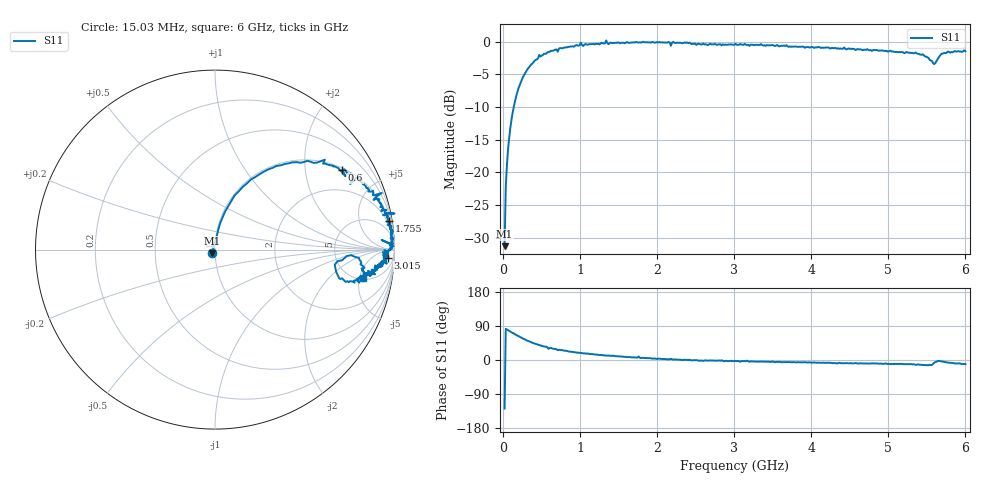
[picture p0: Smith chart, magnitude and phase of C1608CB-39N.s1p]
!	Network	Analyzer	HP8753E.07.74:	Oct	30	2002	Serial	No.	JP38451487
!	Hewlett-Packard
!	7	Sep	2009	9:44:38
!	Frequency	S11
#	HZ	S	RI	R	50
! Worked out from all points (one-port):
!   400 points, 15.03 MHz to 6 GHz, reference 50 ohm
!   lowest |S11| = -31.3 dB at 15.03 MHz (marker M1), VSWR 1.06, Z = 48.3 - j2.08 ohm
!   |S11| at or under -10 dB: start of sweep to 133.9 MHz
!   S11 on the Smith chart (normalised r, x): 15.03 MHz: 0.97, -0.04; 600 MHz: 1.07, +3.15; 1.755 GHz: 1, +12; 3.015 GHz: 20, -26; 6 GHz: 5.27, -5.76
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1.502992e7  -0.0168 -0.0215
3.002985e7  0.0105 0.0768
6.00297e7  0.0293 0.148
1.500292e8  0.132 0.324
3.150284e8  0.392 0.478
4.650277e8  0.612 0.501
6.00027e8  0.709 0.444
7.650262e8  0.798 0.389
1.005025e9  0.929 0.316
1.245024e9  0.926 0.214
1.335023e9  1 0.201
1.365023e9  0.936 0.192
1.515022e9  0.957 0.156
1.725021e9  0.989 0.108
1.755021e9  0.97 0.158
1.785021e9  0.981 0.0857
2.145019e9  0.993 0.0343
2.175019e9  0.928 0.0537
2.205019e9  0.995 0.0182
2.265019e9  0.982 0.019
3.015015e9  0.962 -0.0461
3.765011e9  0.909 -0.0883
4.515007e9  0.873 -0.128
5.265004e9  0.808 -0.159
5.520002e9  0.728 -0.18
5.595002e9  0.667 -0.0846
5.685002e9  0.802 -0.0462
6e9  0.827 -0.159
